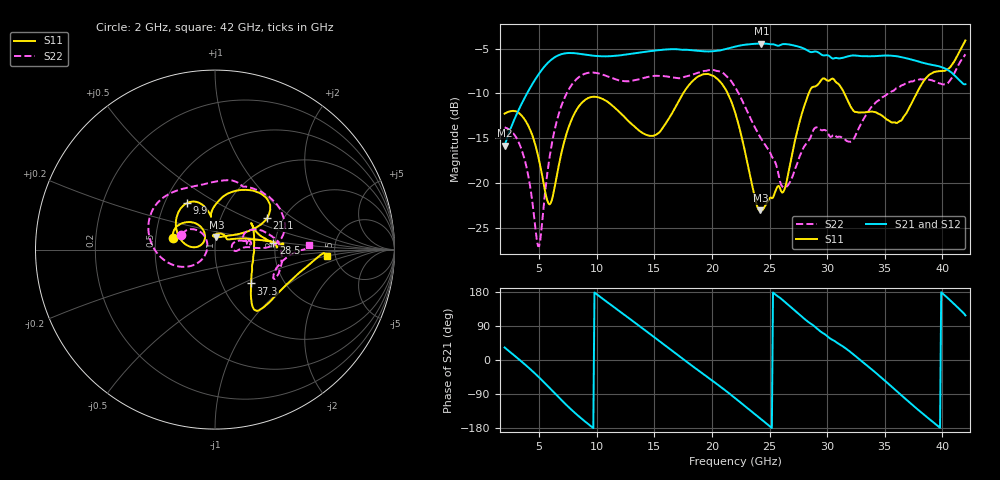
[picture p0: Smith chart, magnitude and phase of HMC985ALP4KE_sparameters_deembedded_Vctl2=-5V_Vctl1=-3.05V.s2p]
!s2p File: Measurements: S11, S21, S12, S22
# GHz S dB R 50.0
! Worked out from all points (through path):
!   401 points, 2 GHz to 42 GHz, reference 50 ohm
!   highest |S21| = -4.45 dB at 24.3 GHz (marker M1); lowest = -15.8 dB at 2 GHz (marker M2)
!   lowest |S11| = -23.0 dB at 24.2 GHz (marker M3), VSWR 1.15, Z = 50.3 + j7.08 ohm
!   |S11| at or under -10 dB: start of sweep to 17.49 GHz; 21.37 GHz to 28.4 GHz (7.037 GHz wide, 28.3 % of centre); 31.49 GHz to 37.77 GHz (6.28 GHz wide, 18.1 % of centre)
!   |S22| runs from -27.0 to -5.6 dB; largest |S21 - S12| = 0.00072
!   S11 on the Smith chart (normalised r, x): 2 GHz: 0.61, +0.08; 9.9 GHz: 0.65, +0.37; 21.1 GHz: 1.66, +0.66; 28.5 GHz: 1.95, +0.16; 37.3 GHz: 1.37, -0.56; 42 GHz: 4.26, -0.47
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2  -12.26 165.3  -15.83 33.1  -15.84 33.1  -13.79 155.9
3.6  -12.66 140.5  -10.85 -7.4  -10.85 -7.4  -16.77 132.3
5  -17.48 121.1  -7.78 -46.1  -7.79 -46.1  -27.03 178.9
6  -22.24 154.0  -6.31 -76.8  -6.31 -76.8  -16.34 -144.8
7.2  -15.26 169.0  -5.55 -113.9  -5.55 -113.8  -10.51 -170.5
8.7  -11.05 139.7  -5.63 -155.2  -5.63 -155.2  -7.97 157.6
9.9  -10.39 121.5  -5.83 175.8  -5.83 175.8  -7.71 138.2
13  -13.39 99.7  -5.59 105.7  -5.59 105.7  -8.61 97.2
15.4  -14.39 97.0  -5.19 50.7  -5.19 50.7  -8.04 73.8
18  -9.08 69.4  -5.16 -9.0  -5.16 -9.0  -8.03 60.5
21.1  -9.38 31.1  -5.09 -78.8  -5.09 -78.7  -7.88 16.2
22  -12.08 28.3  -4.79 -100.5  -4.80 -100.4  -9.28 5.7
24.2  -23.04 83.9  -4.45 -154.5  -4.45 -154.5  -14.89 4.4
24.3  -23.04 88.8  -4.45 -157.0  -4.45 -157.0  -15.10 4.5
26.3  -20.68 37.7  -4.50 153.7  -4.50 153.7  -20.49 8.4
28.5  -9.71 6.6  -5.36 97.5  -5.37 97.5  -15.06 16.1
28.7  -9.31 3.4  -5.39 93.6  -5.40 93.6  -14.41 15.8
32.4  -12.05 24.1  -5.78 11.6  -5.78 11.7  -14.85 27.6
35.4  -13.07 10.1  -5.79 -65.0  -5.79 -64.9  -9.97 14.7
37.3  -11.19 -43.2  -6.23 -115.9  -6.23 -115.8  -8.67 -0.8
39.7  -7.53 -50.1  -6.97 -176.3  -6.98 -176.3  -8.87 -26.0
42  -4.10 -3.1  -8.97 117.7  -8.98 117.7  -5.64 2.9
